| TEXAS INSTRUMENTS INCORPORATED
| Standard Linear and Logic Group
| IBIS Model of SN74CBT16245C
| 16-Bit FET Bus Switch with -2V Undershoot Protection
| This file contains package information for the following:
|  TSSOP 48-pin (DGG) package as [Component] CBT16245C_DGG
|  TVSOP 48-pin (DGV) package as [Component] CBT16245C_DGV
|  SSOP 48-pin (DL) package as [Component] CBT16245C_DL
| This device can be powered at the following Vccs:
|  5 volt Vcc
|  4 volt Vcc
| This file provides unique models under the [Model Selector] for each Vcc.
| For operation at a specific Vcc, select the appropriate model after each
| [Model Selector] keyword.
[IBIS Ver]   3.2
[Comment char]  |_char
[File Name]   sn74cbt16245c.ibs
[File Rev]   1.1 | b_die
[Date]   July 1, 2003
[Source]   Data created from TI-SPICE simulations at TI-SLL.
[Notes]   The following is an IBIS list for the CBT16245C.
   Please contact sllibis@ti.com with questions and
   comments concerning SLL IBIS models.
   - Power-clamp data has been deleted since there is no
   power-clamp diode in the device.
   - Non-monotonic data due to FET characteristics.
[Disclaimer] Property of Texas Instruments Incorporated.  Unauthorized
   reproduction and/or distribution is strictly prohibited.
   This product is protected under copyright law.
   Created  2003, (C) Copyright  2003, Texas Instruments
   Incorporated, All Rights Reserved
   UNLESS THERE IS A SIGNED, WRITTEN AGREEMENT TO THE
   CONTRARY, TEXAS INSTRUMENTS (TI) IS PROVIDING THE IBIS
   MODELS  AND WITHOUT ANY WARRANTY, EXPRESSED OR
   IMPLIED.  TI assumes no liability for:
   1) the accuracy of the IBIS models provided to your
   company;
   2) the proper functioning of these IBIS Models in your
   design or for any resulting applications; or
   3) infringement of patents, copyrights or intellectual
   property rights resulting from your use of these IBIS
   models.
   TI provides IBIS Models as a service to our customers.
   You and your company shall not distribute, sell or give
   these models to anyone else without prior written
   permission from TI.
   TI reserves the right to make changes to our products or
   to discontinue any semiconductor product or service
   without notice, and advises our customers to obtain the
   latest version of relevant information to verify, before
   placing orders, that the information being relied on is
   current.
   Please be aware that your receipt and use of the IBIS
   information provided shall serve as acceptance of these
   terms and conditions.  If you do not accept these terms,
   you should return or destroy the IBIS models and any
   other accompanying information immediately.
| Component CBT16245C_DGG 48-pin TSSOP
[Component]   CBT16245C_DGG
[Manufacturer]   Texas Instruments, Inc.
[Package]
|   typ   min   max
R_pkg   4.400e-02   3.800e-02   5.100e-02
L_pkg   3.019e-09   2.486e-09   4.099e-09
C_pkg   5.070e-13   3.340e-13   8.090e-13
[Pin]   signal_name   model_name   R_pin   L_pin   C_pin
1   NC   NC   4.100e-02   4.017e-09   7.590e-13
2   1B1   CBT16245C_IO   4.200e-02   3.737e-09   7.920e-13
3   1B2   CBT16245C_IO   4.200e-02   3.480e-09   6.610e-13
4   GND   GND   3.800e-02   3.131e-09   5.750e-13
5   1B3   CBT16245C_IO   4.700e-02   3.122e-09   5.660e-13
6   1B4   CBT16245C_IO   4.300e-02   2.948e-09   5.040e-13
7   VCC   POWER   4.500e-02   2.845e-09   3.970e-13
8   1B5   CBT16245C_IO   4.900e-02   2.835e-09   3.940e-13
9   1B6   CBT16245C_IO   4.800e-02   2.715e-09   3.780e-13
10   GND   GND   5.000e-02   2.664e-09   3.630e-13
11   1B7   CBT16245C_IO   5.000e-02   2.585e-09   3.480e-13
12   1B8   CBT16245C_IO   4.900e-02   2.550e-09   3.370e-13
13   2B1   CBT16245C_IO   4.900e-02   2.541e-09   3.360e-13
14   2B2   CBT16245C_IO   5.000e-02   2.574e-09   3.480e-13
15   GND   GND   4.900e-02   2.618e-09   3.590e-13
16   2B3   CBT16245C_IO   4.600e-02   2.671e-09   3.750e-13
17   2B4   CBT16245C_IO   4.500e-02   2.754e-09   3.890e-13
18   VCC   POWER   4.400e-02   2.823e-09   4.500e-13
19   2B5   CBT16245C_IO   4.200e-02   2.968e-09   5.030e-13
20   2B6   CBT16245C_IO   5.100e-02   3.108e-09   5.350e-13
21   GND   GND   4.200e-02   3.175e-09   5.870e-13
22   2B7   CBT16245C_IO   4.100e-02   3.449e-09   6.780e-13
23   2B8   CBT16245C_IO   4.400e-02   3.766e-09   8.040e-13
24   NC   NC   4.300e-02   4.065e-09   7.610e-13
25   2NOE   CBT16245C_IN   4.100e-02   3.994e-09   7.570e-13
26   2A8   CBT16245C_IO   3.900e-02   3.649e-09   7.890e-13
27   2A7   CBT16245C_IO   3.800e-02   3.362e-09   6.600e-13
28   GND   GND   3.800e-02   3.082e-09   5.740e-13
29   2A6   CBT16245C_IO   4.400e-02   2.990e-09   5.220e-13
30   2A5   CBT16245C_IO   4.100e-02   2.917e-09   4.950e-13
31   VCC   POWER   4.300e-02   2.820e-09   4.480e-13
32   2A4   CBT16245C_IO   4.300e-02   2.699e-09   3.850e-13
33   2A3   CBT16245C_IO   4.500e-02   2.628e-09   3.720e-13
34   GND   GND   4.600e-02   2.556e-09   3.560e-13
35   2A2   CBT16245C_IO   4.600e-02   2.495e-09   3.440e-13
36   2A1   CBT16245C_IO   4.700e-02   2.487e-09   3.340e-13
37   1A8   CBT16245C_IO   4.700e-02   2.490e-09   3.350e-13
38   1A7   CBT16245C_IO   4.600e-02   2.486e-09   3.430e-13
39   GND   GND   4.500e-02   2.566e-09   3.560e-13
40   1A6   CBT16245C_IO   4.400e-02   2.639e-09   3.740e-13
41   1A5   CBT16245C_IO   4.300e-02   2.701e-09   3.860e-13
42   VCC   POWER   4.300e-02   2.817e-09   4.500e-13
43   1A4   CBT16245C_IO   4.100e-02   2.935e-09   5.010e-13
44   1A3   CBT16245C_IO   4.700e-02   3.035e-09   5.290e-13
45   GND   GND   4.300e-02   3.171e-09   5.890e-13
46   1A2   CBT16245C_IO   4.000e-02   3.415e-09   6.820e-13
47   1A1   CBT16245C_IO   4.300e-02   3.741e-09   8.090e-13
48   1NOE   CBT16245C_IN   4.400e-02   4.099e-09   7.640e-13
| Component CBT16245C_DGV 48-pin TVSOP
[Component]   CBT16245C_DGV
[Manufacturer]   Texas Instruments, Inc.
[Package]
|   typ   min   max
R_pkg   7.000e-02   4.900e-02   8.500e-02
L_pkg   3.013e-09   2.743e-09   3.408e-09
C_pkg   3.710e-13   2.940e-13   5.110e-13
[Pin]   signal_name   model_name   R_pin   L_pin   C_pin
1   NC   NC   4.900e-02   3.393e-09   4.970e-13
2   1b1   CBT16245C_IO   6.000e-02   3.250e-09   5.020e-13
3   1b2   CBT16245C_IO   7.700e-02   3.310e-09   4.510e-13
4   GND   GND   8.500e-02   3.299e-09   4.040e-13
5   1b3   CBT16245C_IO   8.300e-02   3.136e-09   3.600e-13
6   1b4   CBT16245C_IO   7.700e-02   3.019e-09   3.630e-13
7   VCC   POWER   6.500e-02   2.882e-09   3.490e-13
8   1b5   CBT16245C_IO   6.600e-02   2.829e-09   3.140e-13
9   1b6   CBT16245C_IO   6.700e-02   2.796e-09   3.140e-13
10   GND   GND   6.900e-02   2.754e-09   3.080e-13
11   1b7   CBT16245C_IO   7.000e-02   2.753e-09   3.010e-13
12   1b8   CBT16245C_IO   7.100e-02   2.745e-09   2.940e-13
13   2b1   CBT16245C_IO   7.000e-02   2.744e-09   2.940e-13
14   2b2   CBT16245C_IO   7.000e-02   2.754e-09   3.010e-13
15   GND   GND   6.900e-02   2.754e-09   3.080e-13
16   2b3   CBT16245C_IO   6.700e-02   2.796e-09   3.140e-13
17   2b4   CBT16245C_IO   6.600e-02   2.829e-09   3.140e-13
18   VCC   POWER   6.500e-02   2.883e-09   3.500e-13
19   2b5   CBT16245C_IO   7.500e-02   3.014e-09   3.630e-13
20   2b6   CBT16245C_IO   8.000e-02   3.128e-09   3.580e-13
21   GND   GND   8.400e-02   3.295e-09   4.030e-13
22   2b7   CBT16245C_IO   7.800e-02   3.311e-09   4.520e-13
23   2b8   CBT16245C_IO   6.200e-02   3.259e-09   5.010e-13
24   NC   NC   5.200e-02   3.404e-09   4.960e-13
25   2noe   CBT16245C_IN   5.300e-02   3.397e-09   5.050e-13
26   2a8   CBT16245C_IO   6.200e-02   3.249e-09   5.110e-13
27   2a7   CBT16245C_IO   7.700e-02   3.308e-09   4.530e-13
28   GND   GND   8.200e-02   3.289e-09   4.030e-13
29   2a6   CBT16245C_IO   7.800e-02   3.121e-09   3.590e-13
30   2a5   CBT16245C_IO   7.400e-02   3.010e-09   3.630e-13
31   VCC   POWER   6.500e-02   2.883e-09   3.490e-13
32   2a4   CBT16245C_IO   6.700e-02   2.829e-09   3.140e-13
33   2a3   CBT16245C_IO   6.700e-02   2.795e-09   3.140e-13
34   GND   GND   6.900e-02   2.753e-09   3.070e-13
35   2a2   CBT16245C_IO   7.000e-02   2.753e-09   3.010e-13
36   2a1   CBT16245C_IO   7.000e-02   2.743e-09   2.940e-13
37   1a8   CBT16245C_IO   7.000e-02   2.743e-09   2.940e-13
38   1a7   CBT16245C_IO   7.000e-02   2.753e-09   3.010e-13
39   GND   GND   6.900e-02   2.754e-09   3.070e-13
40   1a6   CBT16245C_IO   6.800e-02   2.797e-09   3.140e-13
41   1a5   CBT16245C_IO   6.700e-02   2.830e-09   3.140e-13
42   VCC   POWER   6.400e-02   2.880e-09   3.490e-13
43   1a4   CBT16245C_IO   7.200e-02   3.004e-09   3.620e-13
44   1a3   CBT16245C_IO   7.800e-02   3.121e-09   3.590e-13
45   GND   GND   8.400e-02   3.296e-09   4.030e-13
46   1a2   CBT16245C_IO   7.700e-02   3.308e-09   4.510e-13
47   1a1   CBT16245C_IO   6.200e-02   3.258e-09   4.990e-13
48   1noe   CBT16245C_IN   5.300e-02   3.408e-09   4.940e-13
| Component CBT16245C_DL 48-pin SSOP
[Component]   CBT16245C_DL
[Manufacturer]   Texas Instruments, Inc.
[Package]
|   typ   min   max
R_pkg   4.800e-02   3.800e-02   5.300e-02
L_pkg   6.046e-09   5.084e-09   7.968e-09
C_pkg   8.130e-13   5.690e-13   1.157e-12
[Pin]   signal_name   model_name   R_pin   L_pin   C_pin
1   NC   NC   4.600e-02   7.968e-09   1.017e-12
2   1b1   CBT16245C_IO   4.400e-02   7.299e-09   1.157e-12
3   1b2   CBT16245C_IO   4.300e-02   6.765e-09   1.058e-12
4   GND   GND   4.100e-02   6.269e-09   9.330e-13
5   1b3   CBT16245C_IO   3.800e-02   5.856e-09   8.290e-13
6   1b4   CBT16245C_IO   4.600e-02   5.802e-09   7.900e-13
7   VCC   POWER   5.000e-02   5.656e-09   7.380e-13
8   1b5   CBT16245C_IO   5.300e-02   5.500e-09   6.430e-13
9   1b6   CBT16245C_IO   5.200e-02   5.304e-09   6.060e-13
10   GND   GND   5.300e-02   5.189e-09   5.830e-13
11   1b7   CBT16245C_IO   5.100e-02   5.084e-09   5.690e-13
12   1b8   CBT16245C_IO   5.300e-02   5.862e-09   8.330e-13
13   2b1   CBT16245C_IO   5.300e-02   5.862e-09   8.330e-13
14   2b2   CBT16245C_IO   5.100e-02   5.084e-09   5.690e-13
15   GND   GND   5.300e-02   5.189e-09   5.830e-13
16   2b3   CBT16245C_IO   5.200e-02   5.304e-09   6.060e-13
17   2b4   CBT16245C_IO   5.300e-02   5.500e-09   6.430e-13
18   VCC   POWER   5.000e-02   5.656e-09   7.380e-13
19   2b5   CBT16245C_IO   4.600e-02   5.802e-09   7.900e-13
20   2b6   CBT16245C_IO   3.800e-02   5.856e-09   8.290e-13
21   GND   GND   4.100e-02   6.269e-09   9.330e-13
22   2b7   CBT16245C_IO   4.300e-02   6.765e-09   1.058e-12
23   2b8   CBT16245C_IO   4.400e-02   7.299e-09   1.157e-12
24   NC   NC   4.600e-02   7.968e-09   1.017e-12
25   2noe   CBT16245C_IN   4.600e-02   7.968e-09   1.017e-12
26   2a8   CBT16245C_IO   4.400e-02   7.299e-09   1.157e-12
27   2a7   CBT16245C_IO   4.300e-02   6.765e-09   1.058e-12
28   GND   GND   4.100e-02   6.269e-09   9.330e-13
29   2a6   CBT16245C_IO   3.800e-02   5.856e-09   8.290e-13
30   2a5   CBT16245C_IO   4.600e-02   5.802e-09   7.900e-13
31   VCC   POWER   5.000e-02   5.656e-09   7.380e-13
32   2a4   CBT16245C_IO   5.300e-02   5.500e-09   6.430e-13
33   2a3   CBT16245C_IO   5.200e-02   5.304e-09   6.060e-13
34   GND   GND   5.300e-02   5.189e-09   5.830e-13
35   2a2   CBT16245C_IO   5.100e-02   5.084e-09   5.690e-13
36   2a1   CBT16245C_IO   5.300e-02   5.862e-09   8.330e-13
37   1a8   CBT16245C_IO   5.300e-02   5.862e-09   8.330e-13
38   1a7   CBT16245C_IO   5.100e-02   5.084e-09   5.690e-13
39   GND   GND   5.300e-02   5.189e-09   5.830e-13
40   1a6   CBT16245C_IO   5.200e-02   5.304e-09   6.060e-13
41   1a5   CBT16245C_IO   5.300e-02   5.500e-09   6.430e-13
42   VCC   POWER   5.000e-02   5.656e-09   7.380e-13
43   1a4   CBT16245C_IO   4.600e-02   5.802e-09   7.900e-13
44   1a3   CBT16245C_IO   3.800e-02   5.856e-09   8.290e-13
45   GND   GND   4.100e-02   6.269e-09   9.330e-13
46   1a2   CBT16245C_IO   4.300e-02   6.765e-09   1.058e-12
47   1a1   CBT16245C_IO   4.400e-02   7.299e-09   1.157e-12
48   1noe   CBT16245C_IN   4.600e-02   7.967e-09   1.017e-12
[Series Switch Groups]
| Function Group States
On  1 /   | 1a1-1a8->1b1-1b8 1noe low
On  2 /   | 2a1-2a8->2b1-2b8 2noe low
On  1 2  /   | enable both
Off 1 2  /   | 1noe high, 2noe high, disable both
[Series Pin Mapping]   pin_2   model_name   function_table_group
37   12   CBT16245C_IO_50_S   1
| 37   12   CBT16245C_IO_40_S   1
38   11   CBT16245C_IO_50_S   1
| 38   11   CBT16245C_IO_40_S   1
40   9   CBT16245C_IO_50_S   1
| 40   9   CBT16245C_IO_40_S   1
41   8   CBT16245C_IO_50_S   1
| 41   8   CBT16245C_IO_40_S   1
43   6   CBT16245C_IO_50_S   1
| 43   6   CBT16245C_IO_40_S   1
44   5   CBT16245C_IO_50_S   1
| 44   5   CBT16245C_IO_40_S   1
46   3   CBT16245C_IO_50_S   1
| 46   3   CBT16245C_IO_40_S   1
47   2   CBT16245C_IO_50_S   1
| 47   2   CBT16245C_IO_40_S   1
26   23   CBT16245C_IO_50_S   2
| 26   23   CBT16245C_IO_40_S   2
27   22   CBT16245C_IO_50_S   2
| 27   22   CBT16245C_IO_40_S   2
29   20   CBT16245C_IO_50_S   2
| 29   20   CBT16245C_IO_40_S   2
30   19   CBT16245C_IO_50_S   2
| 30   19   CBT16245C_IO_40_S   2
32   17   CBT16245C_IO_50_S   2
| 32   17   CBT16245C_IO_40_S   2
33   16   CBT16245C_IO_50_S   2
| 33   16   CBT16245C_IO_40_S   2
35   14   CBT16245C_IO_50_S   2
| 35   14   CBT16245C_IO_40_S   2
36   13   CBT16245C_IO_50_S   2
| 36   13   CBT16245C_IO_40_S   2
| Model CBT16245C_IN
[Model Selector]   CBT16245C_IN
CBT16245C_IN_50   5 volt Vcc
CBT16245C_IN_40   4 volt Vcc
| Model CBT16245C_IO
[Model Selector]   CBT16245C_IO
CBT16245C_IO_50   5 volt Vcc
CBT16245C_IO_40   4 volt Vcc
| Model CBT16245C_IO_S
[Model Selector]   CBT16245C_IO_S
CBT16245C_IO_50_S   5 volt Vcc
CBT16245C_IO_40_S   4 volt Vcc
[Model]   CBT16245C_IO_50_S
Model_type  Series_switch
| variable   typ   min   max
C_comp   0   0   0
[Temperature Range]   40   100   -40
| Ambient temperature   25   85   -40
[Voltage range]   5   4.5   5.5
[On]
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[Off]
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[Model]   CBT16245C_IO_40_S
Model_type  Series_switch
| variable   typ   min   max
C_comp   0   0   0
[Temperature Range]   40   100   -40
| Ambient temperature   25   85   -40
[Voltage range]   4   4   4
[On]
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[Off]
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| Models and submodels in the file (6): CBT16245C_IN_50 (Input), CBT16245C_IN_40 (Input), CBT16245C_IO_50_S (Series_switch), CBT16245C_IO_50 (Terminator), CBT16245C_IO_40_S (Series_switch), CBT16245C_IO_40 (Terminator)
